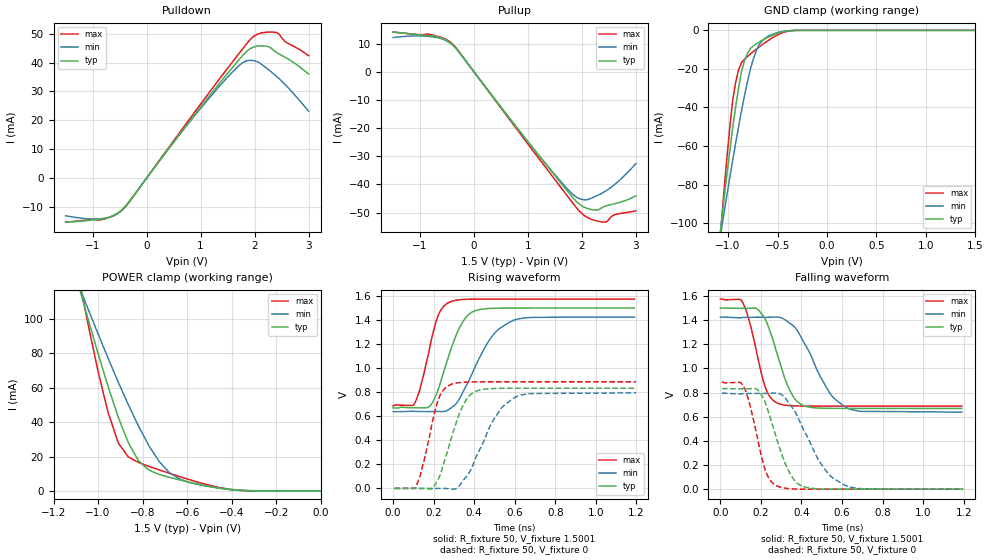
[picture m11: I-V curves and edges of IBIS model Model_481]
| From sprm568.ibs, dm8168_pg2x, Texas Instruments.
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| Model based on original model for BSHTLTCSCDDVGPBFZ
|   Sub model SLOW_10MA_5PER_N_1P5
[model]   Model_481
|[Description]  [1.5V-3-STATE-X-SLOW:10MA, IND, 5%]
|   Slow slew rate (SR[1:0] = "01"), 0.80 * RExt = 1.250 * Iout
|   (I[2:0] = "101"), 10mA nominal with Rext = 50R, ,Industrial
|   temperature range (-40C to 125C, 25C nominal),5% power supply
|   tolerance
|[Input Load]
|[Output Drive] SLOW:10MA
|Voltage   1.5V
|Mode   3-STATE
Model_type   3-state
Polarity   Non-Inverting
Enable   Active-Low
Cref =  15.0000pF
Rref =  100.0000M
Vref =  0V
Vmeas =  0.75005
C_comp   1.5249p   1.4275p   1.6205p
[Model Spec]
[Temperature Range]   25   125   -40
[Voltage Range]   1.5   1.425   1.575
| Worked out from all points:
|   slope of the pulldown table from 0 to 0.225 V, typ, clamps not added: 39.9 ohm
|   slope of the pullup table from 0 to 0.225 V, typ, clamps not added: 39.8 ohm
|   GND clamp passes 1 mA (typ) near -0.47 V on its own axis
|   POWER clamp passes 1 mA (typ) near -0.42 V on its own axis
|   rising waveform, R_fixture 50, V_fixture 1.5001: 20-80 % time 102ps typ, 147ps min, 75.6ps max; typ from 0.669 V to 1.5 V
|   rising waveform, R_fixture 50, V_fixture 0: 20-80 % time 96.4ps typ, 136ps min, 73ps max; typ from 0 V to 0.834 V
|   falling waveform, R_fixture 50, V_fixture 1.5001: 20-80 % time 99.2ps typ, 145ps min, 75.8ps max; typ from 1.5 V to 0.669 V
|   falling waveform, R_fixture 50, V_fixture 0: 20-80 % time 101ps typ, 148ps min, 73.7ps max; typ from 0.833 V to 0 V
[POWER_clamp]
-1.5V     321.7mA    260.6mA    415.9mA
-1.076V   114.2mA    115.8mA    116.9mA
-1.061V   107.2mA    110.9mA    107.1mA
-954.6mV  60.59mA    77.06mA    45.35mA
-909.2mV  42.85mA    63.21mA    27.81mA
-863.7mV  27.9mA     49.99mA    19.69mA
-818.2mV  17.49mA    37.63mA    16.52mA
-772.8mV  12.19mA    26.53mA    14.33mA
-681.9mV  7.985mA    10.89mA    10.33mA
-590.9mV  5.094mA    4.955mA    6.6mA
-363.7mV  298.5uA    465.2uA    297.6uA
0V        1.518nA    24.08nA    367.8pA
[Pulldown]
-1.5V     -15.29mA   -13.07mA   -15.28mA
-772.8mV  -14.07mA   -13.9mA    -14.11mA
-590.9mV  -12.74mA   -12.86mA   -12.82mA
-409.1mV  -10.08mA   -10.11mA   -10.32mA
1.046V    25.68mA    25.17mA    26.75mA
1.591V    38.31mA    36.75mA    40.25mA
1.818V    43.24mA    40.36mA    45.69mA
1.955V    45.18mA    40.77mA    48.64mA
2.091V    45.77mA    39.91mA    50.06mA
2.273V    45.4mA     37.32mA    50.56mA
2.364V    44.07mA    35.93mA    50.51mA
3V        36.04mA    23.14mA    42.4mA
[Pullup]
-1.5V     14.1mA     12.18mA    14.13mA
-818.2mV  12.87mA    12.54mA    13.29mA
-590.9mV  11.83mA    11.72mA    12.11mA
-409.1mV  9.844mA    9.773mA    10.15mA
1.227V    -30.36mA   -30.27mA   -31.43mA
1.727V    -42.29mA   -41.55mA   -44.05mA
1.909V    -46.29mA   -44.65mA   -48.54mA
2.046V    -48.11mA   -45.48mA   -51.1mA
2.227V    -49.12mA   -44.44mA   -52.74mA
2.409V    -47.87mA   -42.71mA   -53.43mA
2.591V    -46.92mA   -40.26mA   -50.87mA
3V        -44.02mA   -32.61mA   -49.35mA
[GND_clamp]
-1.5V     -310.1mA   -250.5mA   -402.5mA
-1.076V   -103.6mA   -106.2mA   -105.2mA
-1.046V   -89.81mA   -96.36mA   -86.02mA
-954.6mV  -51.22mA   -67.87mA   -36.88mA
-924.3mV  -40.08mA   -58.86mA   -27.29mA
-863.7mV  -21.24mA   -41.56mA   -16.73mA
-833.4mV  -15.8mA    -33.75mA   -15.03mA
-772.8mV  -9.345mA   -19.75mA   -12.19mA
-712.2mV  -6.928mA   -10.35mA   -9.704mA
-621.3mV  -4.261mA   -3.896mA   -6.225mA
-409.1mV  -337.1uA   -289.1uA   -618.9uA
1.5V      1.518nA    257.2nA    299pA
[Ramp]
dV/dt_f   0.665312/0.14716328n   0.63012/0.22330251n   0.71/0.11480851n
dV/dt_r 0.67173512/0.14256136n 0.64143768/0.21543312n 0.71245768/0.10990193n
R_load = 50
[Rising Waveform]
R_fixture = 50
V_fixture = 1.5001
V_fixture_min = 1.425
V_fixture_max = 1.575
0s        669.3mV    639.1mV    688.4mV
107.6ps   670.8mV    640.5mV    709.3mV
191.6ps   705.8mV    639.6mV    1.255V
228.7ps   851.7mV    639.5mV    1.461V
277.6ps   1.118V     658.7mV    1.549V
325.3ps   1.327V     738.5mV    1.569V
378.2ps   1.454V     910.6mV    1.574V
476.8ps   1.497V     1.238V     1.575V
575.8ps   1.5V       1.384V     1.575V
1.19ns    1.5V       1.425V     1.575V
[Rising Waveform]
R_fixture = 50
V_fixture = 0
V_fixture_min = 0
V_fixture_max = 0
7.64ps    0V         0V         0V
108.7ps   0V         2.198mV    0V
136.1ps   0V         0V         119.4mV
199.7ps   9.547mV    0V         593.3mV
236.4ps   130.2mV    0V         787.8mV
286.1ps   413.3mV    -5.572mV   864.7mV
388ps     788.4mV    169.9mV    885.5mV
494.1ps   830.9mV    566.4mV    886.6mV
599.7ps   833.2mV    756.4mV    886.8mV
1.198ns   833.5mV    794.6mV    886.9mV
[Falling Waveform]
R_fixture = 50
V_fixture = 1.5001
V_fixture_min = 1.425
V_fixture_max = 1.575
0s        1.499V     1.425V     1.575V
108.7ps   1.498V     1.422V     1.55V
147.3ps   1.499V     1.423V     1.364V
214.2ps   1.429V     1.424V     882.3mV
286.6ps   1.083V     1.425V     709.2mV
332.7ps   855.6mV    1.386V     693.1mV
384.9ps   717.3mV    1.299V     688.9mV
538.7ps   669.3mV    798mV      687.8mV
625.4ps   668.7mV    671.9mV    687.7mV
1.19ns    668.6mV    638.1mV    687.6mV
[Falling Waveform]
R_fixture = 50
V_fixture = 0
V_fixture_min = 0
V_fixture_max = 0
7.64ps    832.6mV    794.3mV    886mV
118.1ps   830.9mV    792.2mV    839.5mV
202.2ps   782.6mV    793.6mV    274mV
235.3ps   647.4mV    793.2mV    102.6mV
287.3ps   366.8mV    793.2mV    20.17mV
334.5ps   158.7mV    721.7mV    5.052mV
390.9ps   35.36mV    562.4mV    0V
509.6ps   0V         177.6mV    0V
605.4ps   0V         40.18mV    0V
1.198ns   0V         0V         0V
